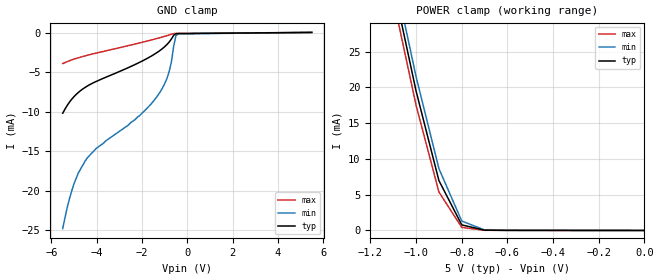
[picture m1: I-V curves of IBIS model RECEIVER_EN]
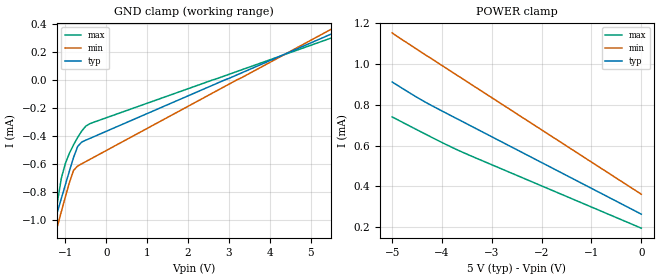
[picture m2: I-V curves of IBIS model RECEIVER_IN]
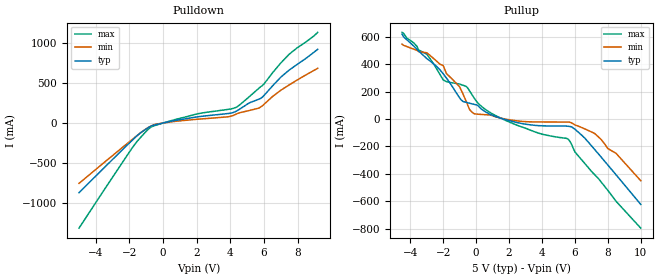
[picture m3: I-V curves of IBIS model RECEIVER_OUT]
|   Texas Instruments Incorporated
|   Data Transmissions Products
|   IBIS Model for TB5R2
|   16DW SOIC Package
[IBIS Ver]   3.2
[Comment char]   |_char
[File name]   tb5r2dw.ibs
[File Rev]   1.0
[Date]   27Jan04
[Source]   File originated at Texas Instruments Incorporated.
   Data Transmission Products Group. All data based on
   Simulation.
[Notes]
[Disclaimer]
(C) Copyright Texas Instruments Incorporated 2004
   All rights reserved
  Texas Instruments Incorporated hereby grants the user of this IBIS
model a non-exclusive, nontransferable license to use this IBIS model
under the following terms.  Before using this IBIS model, the user
should read this license.  If the user does not accept these terms,
the IBIS model should be returned to Texas Instruments within 30 days.
  The user is granted this license only to use the IBIS model and
is not granted rights to sell, load, rent, lease or license the IBIS
model in whole or in part, or in modified form to anyone other than
user.  User may modify the IBIS model to suit its specific applications
but rights to derivative works and such modifications shall belong to
Texas Instruments.
  This IBIS model is provided on an "AS IS" basis and Texas Instruments
makes absolutely no warranty with respect to the information contained
herein.  TEXAS INSTRUMENTS DISCLAIMS AND CUSTOMER WAIVES ALL WARRANTIES,
EXPRESS OR IMPLIED, INCLUDING WARRANTIES OF MERCHANTABILITY OR FITNESS
FOR A PARTICULAR PURPOSE. The entire risk as to quality and performance
is with the Customer. ACCORDINGLY, IN NO EVENT SHALL THE COMPANY BE LIABLE
FOR ANY DAMAGES, WHETHER IN CONTRACT OR TORT,INCLUDING ANY LOST PROFITS
OR OTHER INCIDENTAL, CONSEQUENTIAL, EXEMPLARY, OR PUNITIVE DAMAGES ARISING
OUT OF THE USE OR APPLICATION OF THE IBIS model provided in this package.
Further, Texas Instruments reserves the right to discontinue or make changes
without notice to any product herein to improve reliability, function, or
design. Texas Instruments does not convey any license under patent rights
or any other intellectual property rights, including those of third parties.
Contact Texas Instruments at ATTN:DATA TRANSMISSIONS
[Copyright]   Copyright 2004, Texas Instruments, All Rights Reserved
[Component]   TB5R2
[Manufacturer]  Texas Instruments
[Package]
|   typ   min   max
R_pkg   0.046   0.034   0.057
L_pkg   4.858nH   3.987nH   6.214nH
C_pkg   0.715pF   0.502pF   1.046pF
[Pin]   signal_name   model_name   R_pin   L_pin   C_pin
1   AI(-)   RECEIVER_IN   0.057   6.214nH   1.026pF
2   AI   RECEIVER_IN   0.055   5.236nH   0.818pF
3   AO   RECEIVER_OUT   0.034   3.987nH   0.723pF
4   E1   RECEIVER_EN   0.036   3.996nH   0.726pF
5   BO   RECEIVER_OUT   0.036   3.996nH   0.726pF
6   BI   RECEIVER_IN   0.034   3.987nH   0.704pF
7   BI(-)   RECEIVER_IN   0.055   5.236nH   0.818pF
8   GND   GND   0.057   6.214nH   1.046pF
9   CI(-)   RECEIVER_IN   0.057   6.214nH   0.827pF
10   CI   RECEIVER_IN   0.055   5.236nH   0.597pF
11   CO   RECEIVER_OUT   0.034   3.987nH   0.502pF
12   E2   RECEIVER_EN   0.036   3.996nH   0.505pF
13   DO   RECEIVER_OUT   0.036   3.996nH   0.505pF
14   DI   RECEIVER_IN   0.034   3.987nH   0.502pF
15   DI(-)   RECEIVER_IN   0.055   5.236nH   0.597pF
16   VCC   POWER   0.057   6.214nH   0.827pF
[Diff_pin]   inv_pin   vdiff   tdelay_typ   tdelay_min   tdelay_max
| The 'AI(+) (or 'xI(+)')' and inv_pins, 'AI(-) (or 'xI(-)')', pins
| are Diff_pins
   2   1   100mV   0   0   0
   6   7   100mV   0   0   0
   10   9   100mV   0   0   0
   14   15   100mV   0   0   0
| Models and submodels in the file (3): RECEIVER_EN (Input), RECEIVER_IN (Input), RECEIVER_OUT (3-state)
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|   Receiver Enable Model
[Model]   RECEIVER_EN
Model_type   Input
|Signals   E1,E2
Vinh = 2.4
Vinl = 0.4
|   typ   min   max
C_comp   964fF   924fF   1010fF
|   typ   min   max
[Temperature Range]   25.0   -40   125
[Voltage range]   5.0V   4.5V   5.5V
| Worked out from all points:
|   GND clamp passes 1 mA (typ) near -0.75 V on its own axis
|   POWER clamp passes 1 mA (typ) near -0.80 V on its own axis
[GND_clamp]
| Voltage   I(typ)   I(min)   I(max)
-5.5V     -10.2mA    -24.8mA    -3.93mA
-5.3V     -9.21mA    -22.1mA    -3.68mA
-5V       -8.1mA     -19.1mA    -3.36mA
-4.5V     -6.92mA    -16.2mA    -2.94mA
-4V       -6.16mA    -14.6mA    -2.59mA
-2.1V     -3.76mA    -10.5mA    -1.31mA
-1.5V     -2.83mA    -8.7mA     -876uA
-1.1V     -2.04mA    -7.04mA    -566uA
-800mV    -1.21mA    -4.96mA    -311uA
-700mV    -818uA     -3.71mA    -220uA
-500mV    -158uA     -389uA     -114uA
5.5V      13.6uA     16.5uA     12uA
[Power_clamp]
| Note that the[POWER_clamp]voltage table is referenced to Vcc
| and is calculated using Vtable=Vcc - Vmeasured.
|   Voltage   I(typ)   I(min)   I(max)
-5V       324mA      330mA      323mA
-1.1V     34.4mA     36.4mA     32.4mA
-1V       19.5mA     21.5mA     17.5mA
-900mV    6.98mA     8.65mA     5.38mA
-800mV    782uA      1.32mA     431uA
-700mV    41.2uA     71.3uA     26.6uA
0V        1.02uA     633nA      1.75uA
|   Receiver Input Model
[Model]   RECEIVER_IN
Model_type   Input
|Signals   AI,AI(-),BI,BI(-),CI,CI(-),DI,DI(-)
Vinh = 3.3
Vinl = 3.1
|   typ   min   max
C_comp   61.4fF   61.4fF   61.4fF
|   typ   min   max
[Temperature Range]   25.0   -40   125
[Voltage range]   5.0V   4.5V   5.5V
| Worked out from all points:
|   GND clamp passes 1 mA (typ) near -1.25 V on its own axis
[GND_clamp]
| Voltage   I(typ)   I(min)   I(max)
-5.5V     -73.88mA   -133.6mA   -75.47mA
-1.4V     -1.14mA    -1.266mA   -1.771mA
-1.3V     -1.044mA   -1.158mA   -1.213mA
-1.2V     -946.3uA   -1.05mA    -884.2uA
-1.1V     -847.6uA   -941.8uA   -702.9uA
-1V       -748.1uA   -834.3uA   -596.2uA
-900mV    -648.8uA   -730.7uA   -522.6uA
-800mV    -553.4uA   -645.9uA   -463.3uA
-700mV    -475.5uA   -614.8uA   -411uA
-600mV    -443.7uA   -598.8uA   -364.9uA
-500mV    -430.2uA   -583uA     -330.1uA
5.5V      327.2uA    361.6uA    298.8uA
[Power_clamp]
| Note that the[POWER_clamp]voltage table is referenced to Vcc
| and is calculated using Vtable=Vcc - Vmeasured.
|   Voltage   I(typ)   I(min)   I(max)
-5V       912.2uA    1.153mA    740.9uA
-4.4V     822.4uA    1.056mA    665uA
-3.6V     719.4uA    929.9uA    569uA
0V        263.9uA    361.6uA    195.2uA
|   Receiver Output Model
[Model]   RECEIVER_OUT
Model_type   3-state
| Signals   AO,BO,CO,DO
Vmeas = 1.5V   |Reference voltage for timing measurements
Cref = 10pF   |Timing specification test load capacitance value
| variable   typ   min   max
C_comp   967fF   940fF   1007fF
|   typ   min   max
[Temperature Range]   25.0   -40   125
[Voltage range]   5.0V   4.5V   5.5V
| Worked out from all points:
|   slope of the pulldown table from 0 to 0.75 V, typ, clamps not added: 23 ohm
|   slope of the pullup table from 0 to 0.75 V, typ, clamps not added: 11.8 ohm
[Pulldown]
|   Voltage   I(typ)   I(min)   I(max)
-5V       -868mA     -752mA     -1.31A
-1.8V     -208mA     -199mA     -300mA
-800mV    -47.4mA    -46.5mA    -63.1mA
-300mV    -14.3mA    -9.76mA    -19.3mA
1.8V      69.3mA     42.6mA     102mA
3.9V      119mA      78.8mA     171mA
4.4V      153mA      116mA      202mA
5.7V      298mA      187mA      433mA
6V        342mA      232mA      486mA
7V        571mA      408mA      748mA
7.5V      660mA      475mA      857mA
9.2V      919mA      682mA      1.13A
[Pullup]
|   Voltage   I(typ)   I(min)   I(max)
| Note that the[Pullup]voltage table is referenced to Vcc
| and is calculated using Vtable=Vcc - Vmeasured.
-4.5V     620mA      547mA      633mA
-3V       442mA      484mA      474mA
-2V       331mA      390mA      286mA
-1.8V     299mA      332mA      273mA
-900mV    139mA      209mA      251mA
-400mV    116mA      70mA       206mA
-100mV    107mA      38.7mA     150mA
1.9V      -7.45mA    -2.48mA    -15.5mA
5.6V      -52.7mA    -21.7mA    -148mA
6V        -74.1mA    -42.5mA    -240mA
7.2V      -222mA     -105mA     -406mA
10V       -623mA     -450mA     -796mA
[Ramp]
|   typ   min   max
dV/dt_r   1.973V/1573ps   1.912V/2557ps   1.852V/1318ps
dV/dt_f   1.998V/1311ps   1.966V/1883ps   2.013V/994ps
R_load = 2000
